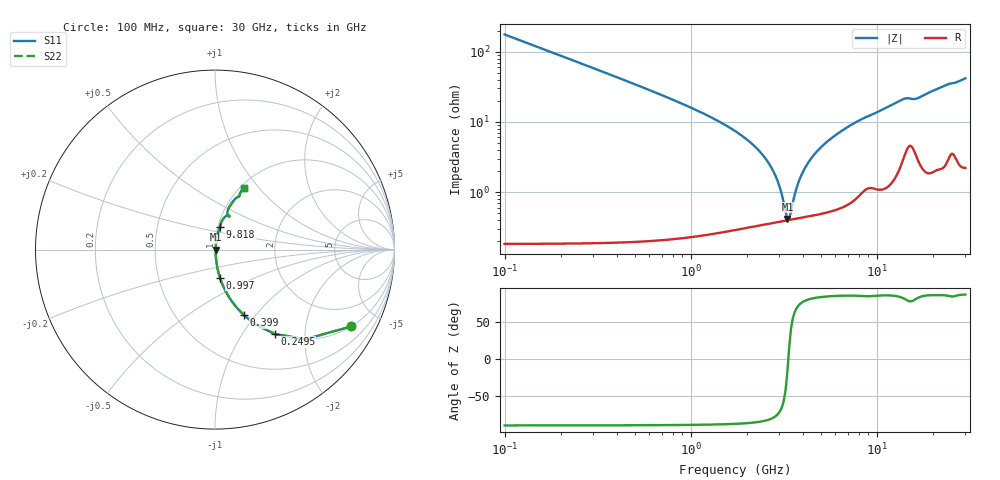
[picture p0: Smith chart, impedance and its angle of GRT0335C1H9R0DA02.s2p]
!Murata Part Number: GRT0335C1H9R0DA02
!These Parameters are Measured in Series Mode Connection
!Data Generated on Jun 19, 2026
!  o--ll--o
!Port1  Port2
!  o------o
!Operation Temp=25[degC], DC Bias Voltage=0[V]
!Freq. Start=100[MHz] Stop=30[GHz] 401[Steps]
# Hz S RI R 50
!Freq.(Hz) S11(Real) S11(Imag) S21(Real) S21(Imag) S12(Real) S12(Imag) S22(Real) S22(Imag)
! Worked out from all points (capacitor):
!   401 points, 100 MHz to 30 GHz, reference 50 ohm
!   read as one part in series: C = 9 pF near 249.5 MHz
!   lowest |Z| = 412 mohm at 3.314 GHz (marker M1)
!   series resonance near 3.352 GHz, so ESL is about 250 pH
!   S11 on the Smith chart (normalised r, x): 100 MHz: 1.00, -3.53; 249.5 MHz: 1.00, -1.41; 399 MHz: 1.00, -0.87; 997 MHz: 1.00, -0.32; 9.818 GHz: 1.02, +0.27; 30 GHz: 1.04, +0.84
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1e8  0.7571 -0.4283  0.2429 0.4283  0.2429 0.4283  0.7571 -0.4283
2.495e8  0.3322 -0.4697  0.6678 0.4697  0.6678 0.4697  0.3322 -0.4697
3.99e8  0.1612 -0.3656  0.8388 0.3656  0.8388 0.3656  0.1612 -0.3656
6.2325e8  0.0712 -0.2535  0.9288 0.2535  0.9288 0.2535  0.0712 -0.2535
9.97e8  0.0274 -0.1563  0.9726 0.1563  0.9726 0.1563  0.0274 -0.1563
2.56675e9  0.00426 -0.028  0.9957 0.028  0.9957 0.028  0.00426 -0.028
2.86575e9  0.00393 -0.0163  0.9961 0.0163  0.9961 0.0163  0.00393 -0.0163
3.2395e9  0.0039 -0.00352  0.9961 0.00352  0.9961 0.00352  0.0039 -0.00352
3.31425e9  0.00393 -0.00116  0.9961 0.00116  0.9961 0.00116  0.00393 -0.00116
3.46375e9  0.00403 0.0034  0.996 -0.0034  0.996 -0.0034  0.00403 0.0034
3.76275e9  0.00432 0.012  0.9957 -0.012  0.9957 -0.012  0.00432 0.012
4.06175e9  0.00473 0.0199  0.9953 -0.0199  0.9953 -0.0199  0.00473 0.0199
4.51025e9  0.00554 0.0311  0.9945 -0.0311  0.9945 -0.0311  0.00554 0.0311
5.10825e9  0.00691 0.0447  0.9931 -0.0447  0.9931 -0.0447  0.00691 0.0447
7.05175e9  0.0138 0.0839  0.9862 -0.0839  0.9862 -0.0839  0.0138 0.0839
9.8175e9  0.0277 0.1278  0.9723 -0.1278  0.9723 -0.1278  0.0277 0.1278
1.01165e10  0.0289 0.1327  0.9711 -0.1327  0.9711 -0.1327  0.0289 0.1327
1.34055e10  0.0587 0.1854  0.9413 -0.1854  0.9413 -0.1854  0.0587 0.1854
1.505e10  0.0811 0.1859  0.9189 -0.1859  0.9189 -0.1859  0.0811 0.1859
2.005825e10  0.0866 0.2488  0.9134 -0.2488  0.9134 -0.2488  0.0866 0.2488
2.50665e10  0.1335 0.2949  0.8665 -0.2949  0.8665 -0.2949  0.1335 0.2949
3e10  0.162 0.343  0.838 -0.343  0.838 -0.343  0.162 0.343
